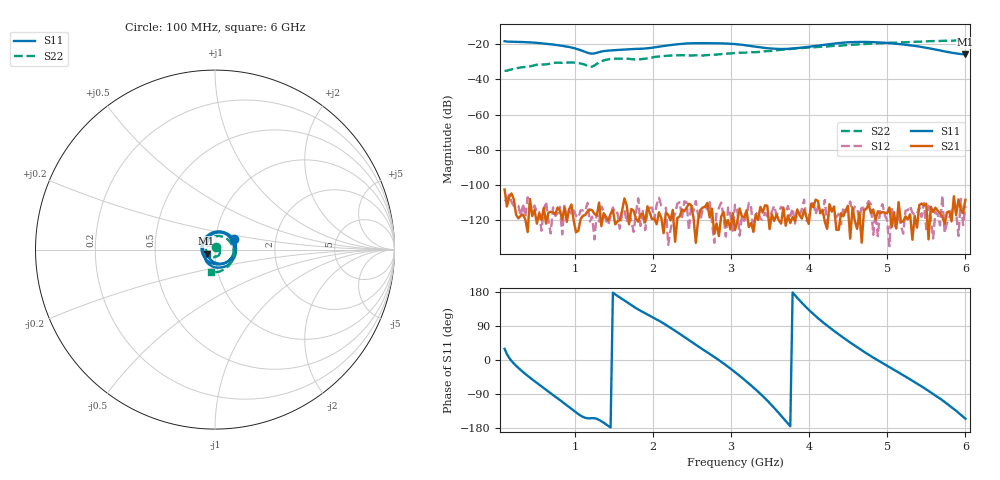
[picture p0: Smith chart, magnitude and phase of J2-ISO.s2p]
!Agilent Technologies,E8364B,MY43040379,A.07.50.67
!Agilent E8364B: A.07.50.67
!Date: Tuesday, March 24, 2026 11:36:23
!Correction: S11(Full 2 Port(1,2))
!S21(Full 2 Port(1,2))
!S12(Full 2 Port(1,2))
!S22(Full 2 Port(1,2))
!S2P File: Measurements: S11, S21, S12, S22:
# Hz S  dB  R 50
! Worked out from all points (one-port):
!   201 points, 100 MHz to 6 GHz, reference 50 ohm
!   lowest |S11| = -25.8 dB at 6 GHz (marker M1), VSWR 1.11, Z = 45.5 - j1.99 ohm
!   |S11| at or under -10 dB: start of sweep to end of sweep
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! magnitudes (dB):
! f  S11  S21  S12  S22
! 100 MHz  -18.3  -102.6  -109.4  -35.2
! 513 MHz  -19.2  -122.0  -115.9  -31.7
! 749 MHz  -20.4  -116.6  -117.7  -30.6
! 985 MHz  -22.2  -120.5  -114.5  -30.4
! 1.103 GHz  -23.9  -117.6  -114.5  -31.3
! 1.192 GHz  -25.3  -114.0  -120.9  -32.8
! 1.221 GHz  -25.4  -114.4  -118.0  -32.8
! 1.339 GHz  -24.2  -123.5  -112.2  -29.7
! 1.427 GHz  -23.7  -120.3  -122.8  -28.6
! 1.634 GHz  -23.1  -107.7  -114.3  -28.2
! 1.782 GHz  -22.7  -119.1  -116.0  -28.7
! 2.076 GHz  -21.5  -115.5  -107.4  -27.0
! 2.46 GHz  -19.5  -110.7  -125.9  -26.4
! 2.637 GHz  -19.4  -112.9  -113.7  -26.4
! 3.05 GHz  -19.9  -125.8  -111.3  -25.0
! 3.611 GHz  -22.7  -120.1  -115.4  -23.3
! 3.817 GHz  -22.4  -120.6  -122.0  -22.5
! 4.053 GHz  -21.1  -112.7  -109.0  -21.8
! 4.554 GHz  -18.8  -112.8  -115.7  -20.4
! 5.027 GHz  -19.4  -112.9  -134.9  -19.2
! 5.38 GHz  -21.1  -124.3  -116.4  -18.5
! 6 GHz  -25.8  -108.4  -111.9  -17.9
